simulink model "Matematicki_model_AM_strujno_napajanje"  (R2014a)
settings: Solver=ode3  StartTime=0.0  StopTime=Tfinalno  FixedStep=Tsim  RelTol=1e-3
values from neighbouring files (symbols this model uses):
  A1 = [-1/Tr 0; 0 -1/Tr]    [Matematicki_model_AM_strujno_napajanje_parametri.m]
  A2 = [0 1; -1 0]    [Matematicki_model_AM_strujno_napajanje_parametri.m]
  A3 = [0 -1; 1 0]    [Matematicki_model_AM_strujno_napajanje_parametri.m]
  Am = [-Kfv*p/J -Kel*p/J; 1 0]    [Matematicki_model_AM_strujno_napajanje_parametri.m]
  B = [Lm/Tr 0; 0 Lm/Tr]    [Matematicki_model_AM_strujno_napajanje_parametri.m]
  Bm = [p/J -p/J; 0 0]    [Matematicki_model_AM_strujno_napajanje_parametri.m]
  Im = sqrt(2)*Ieff    [Matematicki_model_AM_strujno_napajanje_parametri.m]
  Kp = -5.0    (= -5)    [Matematicki_model_AM_strujno_napajanje_parametri.m]
  Lm = 0.422    [Matematicki_model_AM_strujno_napajanje_parametri.m]
  Lr = Lxr+Lm    (= 0.462)    [Matematicki_model_AM_strujno_napajanje_parametri.m]
  Lsigma = Ls*sigm    (= 0.0765367965368)    [Matematicki_model_AM_strujno_napajanje_parametri.m]
  Mopt = 1    [Matematicki_model_AM_strujno_napajanje_parametri.m]
  p = 2    [Matematicki_model_AM_strujno_napajanje_parametri.m]
  Rs = 10.0    (= 10)    [Matematicki_model_AM_strujno_napajanje_parametri.m]
  Tn = 10*Tr    (= 0.733333333333)    [Matematicki_model_AM_strujno_napajanje_parametri.m]
  topt = 0    [Matematicki_model_AM_strujno_napajanje_parametri.m]
  TROUGAO_ZVEZDA = 0    [Matematicki_model_AM_strujno_napajanje_parametri.m]
  Tsim = Tpwm/16    (= 3.125e-06)    [Matematicki_model_AM_strujno_napajanje_parametri.m]
  wk = 1/Tr    (= 13.6363636364)    [Matematicki_model_AM_strujno_napajanje_parametri.m]
  wref = ws    [Matematicki_model_AM_strujno_napajanje_parametri.m]
  ws = 2*pi()*fs    [Matematicki_model_AM_strujno_napajanje_parametri.m]
libraries: simulink x1

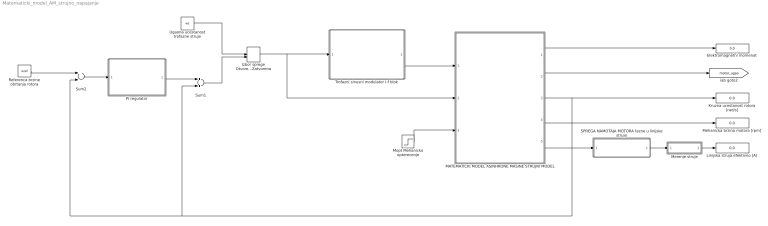
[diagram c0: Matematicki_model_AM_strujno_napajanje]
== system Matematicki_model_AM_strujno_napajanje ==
  Elektromagnetni momenat : Display
  Izbor sprege Otvorena / Zatvorena : ManualSwitch  CurrentSetting=0
  Kruzna ucestanost rotora [rad/s] : Display
  Linijska struja efektivno [A] : Display
  MATEMATICKI MODEL ASINHRONE MASINE STRUJNI MODEL : Subsystem
  Mehanicka brzina motora [rpm] : Display
  Merenje struje : Subsystem
  Mopt Mehanicko opterecenje : Step  Time=topt  After=Mopt  SampleTime=Tsim
  PI regulator : Subsystem
  Referenca brzine obrtanja rotora : Constant  Value=wref  SampleTime=Tsim
  SPREGA NAMOTAJA MOTORA fazne u linijske struje : Subsystem
  Sum1 : Sum  SampleTime=Tsim
  Sum2 : Sum  Inputs=+-  SampleTime=Tsim
  Trofazni sinusni modulator I-f blok : Subsystem
  Ugaona ucestanost trofazne struje : Constant  Value=ws  SampleTime=Tsim
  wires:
  Merenje struje/1(Is_eff) -> Linijska struja efektivno [A]/1
  SPREGA NAMOTAJA MOTORA fazne u linijske struje/1("Is_abc invertor ") -> Merenje struje/1(Is_abc)
  MATEMATICKI MODEL ASINHRONE MASINE STRUJNI MODEL/5(" Is_abc ") -> SPREGA NAMOTAJA MOTORA fazne u linijske struje/1(Is_abc fazno)
  MATEMATICKI MODEL ASINHRONE MASINE STRUJNI MODEL/4(Brzina meh [o/min]) -> Mehanicka brzina motora [rpm]/1
  MATEMATICKI MODEL ASINHRONE MASINE STRUJNI MODEL/1(M_el) -> Elektromagnetni momenat/1
  MATEMATICKI MODEL ASINHRONE MASINE STRUJNI MODEL/3(wr_el) -> Kruzna ucestanost rotora [rad/s]/1, Sum2/2, Sum1/2
  Referenca brzine obrtanja rotora/1 -> Sum2/1
  Sum2/1 -> PI regulator/1(e)
  PI regulator/1(wk) -> Sum1/1
  Trofazni sinusni modulator I-f blok/1(PWM) -> MATEMATICKI MODEL ASINHRONE MASINE STRUJNI MODEL/1(Is_abc)
  Izbor sprege Otvorena / Zatvorena/1 -> MATEMATICKI MODEL ASINHRONE MASINE STRUJNI MODEL/2(W_dq), Trofazni sinusni modulator I-f blok/1(ws)
  Sum1/1 -> Izbor sprege Otvorena / Zatvorena/2
  Ugaona ucestanost trofazne struje/1 -> Izbor sprege Otvorena / Zatvorena/1
  MATEMATICKI MODEL ASINHRONE MASINE STRUJNI MODEL/2(ugao rot_el) -> [motor_ugao]
  Mopt Mehanicko opterecenje/1 -> MATEMATICKI MODEL ASINHRONE MASINE STRUJNI MODEL/3(Mopt)

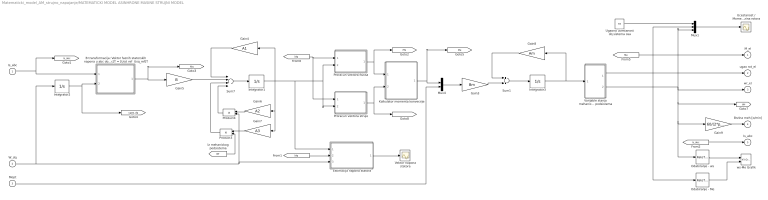
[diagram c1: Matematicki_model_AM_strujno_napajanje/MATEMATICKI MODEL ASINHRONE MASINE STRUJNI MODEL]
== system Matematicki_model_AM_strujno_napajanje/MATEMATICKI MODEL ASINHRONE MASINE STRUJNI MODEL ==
  Is_abc : Inport
  W_dq : Inport  Port=2
  Mopt : Inport  Port=3
  B transformacija: Vektor faznih statorskih napona u abc domenu u vektor napona u dq referentnom sistemu - [Usa  Usb Usc]T = [Usd_ref  Usq_ref]T : Subsystem
  Estimacija napona statora : Subsystem
  Gain3 : Gain  Gain=Bm  Multiplication=Matrix(K*u) (u vector)  SampleTime=Tsim
  Gain4 : Gain  Gain=A1  Multiplication=Matrix(K*u) (u vector)  SampleTime=Tsim
  Gain5 : Gain  Gain=B  Multiplication=Matrix(K*u) (u vector)  SampleTime=Tsim
  Gain6 : Gain  Gain=A2  Multiplication=Matrix(K*u) (u vector)  SampleTime=Tsim
  Gain7 : Gain  Gain=A3  Multiplication=Matrix(K*u) (u vector)  SampleTime=Tsim
  Gain8 : Gain  Gain=Am  Multiplication=Matrix(K*u) (u vector)  SampleTime=Tsim
  Gain9 : Gain  Gain=60/(2*pi()*p)  SampleTime=Tsim
  Integrator1 : Integrator  InitialCondition=[0,0]
  Integrator2 : Integrator
  Integrator3 : Integrator  InitialCondition=[0,0]
  Kalkulator momenta konverzije : Subsystem
  Mux1 : Mux  Inputs=3
  Mux4 : Mux  Inputs=2
  Odabiranje - Me : RateTransition  OutPortSampleTime=100*Tsim
  Odabiranje - ws : RateTransition  OutPortSampleTime=100*Tsim
  Product3 : Product  SampleTime=Tsim
  Product4 : Product  SampleTime=Tsim
  Proracun vektora fluksa : Subsystem
  Proracun vektora struje : Subsystem
  Sum1 : Sum  SampleTime=Tsim
  Sum7 : Sum  Inputs=++++  SampleTime=Tsim
  Ucestanost / Momenat / Brzina rotora : Scope
  Ugaona ucestanost dq sistema osa : Constant  Value=ws  SampleTime=Tsim
  Varijable stanja mehanickog podsistema : Subsystem
  Vektor napona statora : Scope
  ws-Me Grafik : simulink/Sinks/XY Graph  xmin=-400  xmax=400  ymin=-5  ymax=5  st=100*Tsim
  M_el : Outport  InitialOutput=0
  ugao rot_el : Outport  Port=2  InitialOutput=0
  wr_el : Outport  Port=3  InitialOutput=0
  Brzina meh [o/min] : Outport  Port=4  InitialOutput=0
  " Is_abc " : Outport  Port=5  InitialOutput=0
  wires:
  Odabiranje - Me/1 -> ws-Me Grafik/2
  Odabiranje - ws/1 -> ws-Me Grafik/1
  Mux1/1 -> Ucestanost / Momenat / Brzina rotora/1
  [Is_abc] -> " Is_abc "/1
  Integrator3/1 -> Gain8/1, Varijable stanja mehanickog podsistema/1(X2)
  Gain8/1 -> Sum1/1
  Sum1/1 -> Integrator3/1
  Gain3/1 -> Sum1/2
  Mux4/1 -> Gain3/1
  Gain9/1 -> Brzina meh [o/min]/1
  Varijable stanja mehanickog podsistema/2(w) -> Odabiranje - ws/1, Gain9/1, [Wr], Mux1/3, wr_el/1
  Varijable stanja mehanickog podsistema/1(theta) -> ugao rot_el/1
  [Me] -> Odabiranje - Me/1, Mux1/2, M_el/1
  Mopt/1 -> Mux4/2
  Kalkulator momenta konverzije/1(Me) -> Mux4/1, [Me]
  Proracun vektora struje/1(I) -> Kalkulator momenta konverzije/2(I), [I]
  Proracun vektora fluksa/1(PSI) -> Kalkulator momenta konverzije/1(PSI), [PSI]
  Product4/1 -> Sum7/4
  W_dq/1 -> Product4/2, Estimacija napona statora/3(wdq), Integrator2/1
  Gain5/1 -> Sum7/2
  Gain4/1 -> Sum7/1
  Sum7/1 -> Integrator1/1
  Gain6/1 -> Product4/1
  Gain7/1 -> Product3/1
  Product3/1 -> Sum7/3
  [Wr] -> Product3/2
  Is_abc/1 -> [Is_abc], B transformacija: Vektor faznih statorskih napona u abc domenu u vektor napona u dq referentnom sistemu - [Usa  Usb Usc]T = [Usd_ref  Usq_ref]T/1(Is_abc)
  [Idq] -> Proracun vektora fluksa/1(Is), Proracun vektora struje/1(Is)
  Estimacija napona statora/1(Vs) -> Vektor napona statora/1
  Integrator2/1 -> [ugao_dq], B transformacija: Vektor faznih statorskih napona u abc domenu u vektor napona u dq referentnom sistemu - [Usa  Usb Usc]T = [Usd_ref  Usq_ref]T/2(ugao_dq)
  B transformacija: Vektor faznih statorskih napona u abc domenu u vektor napona u dq referentnom sistemu - [Usa  Usb Usc]T = [Usd_ref  Usq_ref]T/1(Is_dq) -> Gain5/1, [Idq]
  [Idq] -> Estimacija napona statora/2(Is)
  Integrator1/1 -> Gain6/1, Gain7/1, Estimacija napona statora/1(PSIr), Proracun vektora struje/2(PSIr), Proracun vektora fluksa/2(PSIr), Gain4/1
  Ugaona ucestanost dq sistema osa/1 -> Mux1/1

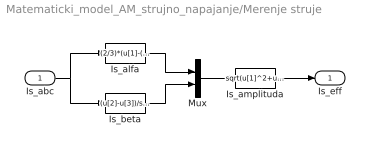
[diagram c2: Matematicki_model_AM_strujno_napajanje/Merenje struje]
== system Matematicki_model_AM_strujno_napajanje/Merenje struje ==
  Is_abc : Inport
  Is_alfa : Fcn  Expr=(2/3)*(u[1]-(u[2]+u[3])/2)  SampleTime=Tsim
  Is_amplituda : Fcn  Expr=sqrt(u[1]^2+u[2]^2)/sqrt(2)  SampleTime=Tsim
  Is_beta : Fcn  Expr=(u[2]-u[3])/sqrt(3)  SampleTime=Tsim
  Mux : Mux  Inputs=2
  Is_eff : Outport
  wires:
  Is_abc/1 -> Is_beta/1, Is_alfa/1
  Is_alfa/1 -> Mux/1
  Is_beta/1 -> Mux/2
  Mux/1 -> Is_amplituda/1
  Is_amplituda/1 -> Is_eff/1

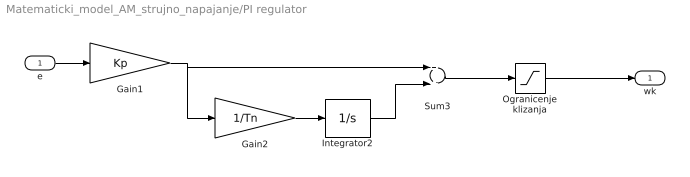
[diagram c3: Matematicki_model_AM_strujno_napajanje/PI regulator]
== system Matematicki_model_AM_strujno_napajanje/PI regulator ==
  e : Inport
  Gain1 : Gain  Gain=Kp  SampleTime=Tsim
  Gain2 : Gain  Gain=1/Tn  SampleTime=Tsim
  Integrator2 : Integrator  InitialCondition=[0]
  Ogranicenje klizanja : Saturate  UpperLimit=inf  LowerLimit=wk  SampleTime=Tsim
  Sum3 : Sum  SampleTime=Tsim
  wk : Outport
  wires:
  Gain1/1 -> Sum3/1, Gain2/1
  e/1 -> Gain1/1
  Sum3/1 -> Ogranicenje klizanja/1
  Integrator2/1 -> Sum3/2
  Gain2/1 -> Integrator2/1
  Ogranicenje klizanja/1 -> wk/1

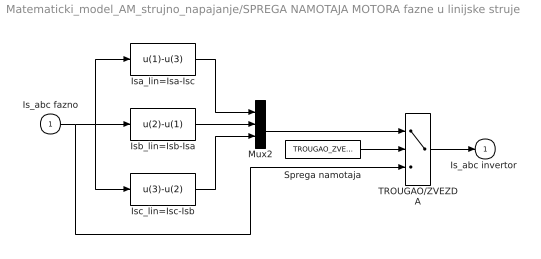
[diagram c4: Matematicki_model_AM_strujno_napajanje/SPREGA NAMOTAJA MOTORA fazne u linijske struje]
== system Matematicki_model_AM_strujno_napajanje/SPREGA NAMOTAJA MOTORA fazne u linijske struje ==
  Is_abc fazno : Inport
  Isa_lin=Isa-Isc : Fcn  Expr=u(1)-u(3)  SampleTime=Tsim
  Isb_lin=Isb-Isa : Fcn  Expr=u(2)-u(1)  SampleTime=Tsim
  Isc_lin=Isc-Isb : Fcn  Expr=u(3)-u(2)  SampleTime=Tsim
  Mux2 : Mux  Inputs=3
  Sprega namotaja : Constant  Value=TROUGAO_ZVEZDA
  TROUGAO/ZVEZDA : Switch  Threshold=0.1  SampleTime=Tsim
  "Is_abc invertor " : Outport  InitialOutput=0
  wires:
  Sprega namotaja/1 -> TROUGAO/ZVEZDA/2
  Mux2/1 -> TROUGAO/ZVEZDA/1
  TROUGAO/ZVEZDA/1 -> "Is_abc invertor "/1
  Is_abc fazno/1 -> TROUGAO/ZVEZDA/3, Isa_lin=Isa-Isc/1, Isb_lin=Isb-Isa/1, Isc_lin=Isc-Isb/1
  Isa_lin=Isa-Isc/1 -> Mux2/1
  Isb_lin=Isb-Isa/1 -> Mux2/2
  Isc_lin=Isc-Isb/1 -> Mux2/3

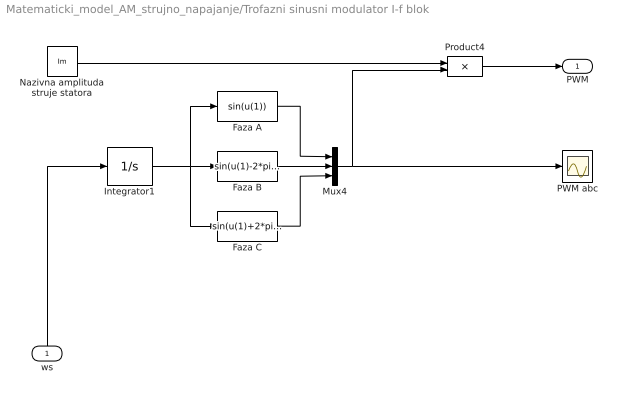
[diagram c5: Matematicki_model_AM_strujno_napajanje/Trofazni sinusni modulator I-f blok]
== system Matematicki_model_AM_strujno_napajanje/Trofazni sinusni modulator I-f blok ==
  ws : Inport
  Faza A : Fcn  Expr=sin(u(1))  SampleTime=Tsim
  Faza B : Fcn  Expr=sin(u(1)-2*pi()/3)  SampleTime=Tsim
  Faza C : Fcn  Expr=sin(u(1)+2*pi()/3)  SampleTime=Tsim
  Integrator1 : Integrator  InitialCondition=[0]
  Mux4 : Mux  Inputs=3
  Nazivna amplituda struje statora : Constant  Value=Im  SampleTime=Tsim
  PWM abc : Scope
  Product4 : Product  SampleTime=Tsim
  PWM : Outport
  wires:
  Faza B/1 -> Mux4/2
  Faza A/1 -> Mux4/1
  Faza C/1 -> Mux4/3
  Mux4/1 -> Product4/2, PWM abc/1
  Nazivna amplituda struje statora/1 -> Product4/1
  Product4/1 -> PWM/1
  ws/1 -> Integrator1/1
  Integrator1/1 -> Faza C/1, Faza B/1, Faza A/1

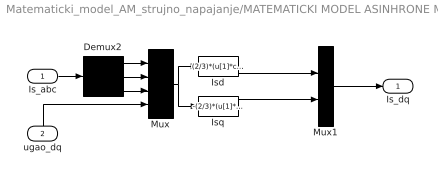
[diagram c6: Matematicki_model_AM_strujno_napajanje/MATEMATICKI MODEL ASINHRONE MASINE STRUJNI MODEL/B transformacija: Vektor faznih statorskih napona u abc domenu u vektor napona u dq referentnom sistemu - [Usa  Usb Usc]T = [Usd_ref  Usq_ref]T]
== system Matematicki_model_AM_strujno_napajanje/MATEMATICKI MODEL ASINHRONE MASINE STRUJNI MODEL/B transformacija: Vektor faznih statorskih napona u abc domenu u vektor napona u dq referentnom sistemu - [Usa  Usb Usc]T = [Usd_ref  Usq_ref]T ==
  Is_abc : Inport
  ugao_dq : Inport  Port=2
  Demux2 : Demux  Outputs=3
  Isd : Fcn  Expr=(2/3)*(u[1]*cos(u[4])+u[2]*cos(u[4]-2*pi/3)+u[3]*cos(u[4]-4*pi/3))  SampleTime=Tsim
  Isq : Fcn  Expr=-(2/3)*(u[1]*sin(u[4])+u[2]*sin(u[4]-2*pi/3)+u[3]*sin(u[4]-4*pi/3))  SampleTime=Tsim
  Mux : Mux
  Mux1 : Mux  Inputs=2
  Is_dq : Outport
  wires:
  Mux1/1 -> Is_dq/1
  Is_abc/1 -> Demux2/1
  ugao_dq/1 -> Mux/4
  Demux2/1 -> Mux/1
  Demux2/3 -> Mux/3
  Demux2/2 -> Mux/2
  Mux/1 -> Isd/1, Isq/1
  Isq/1 -> Mux1/2
  Isd/1 -> Mux1/1

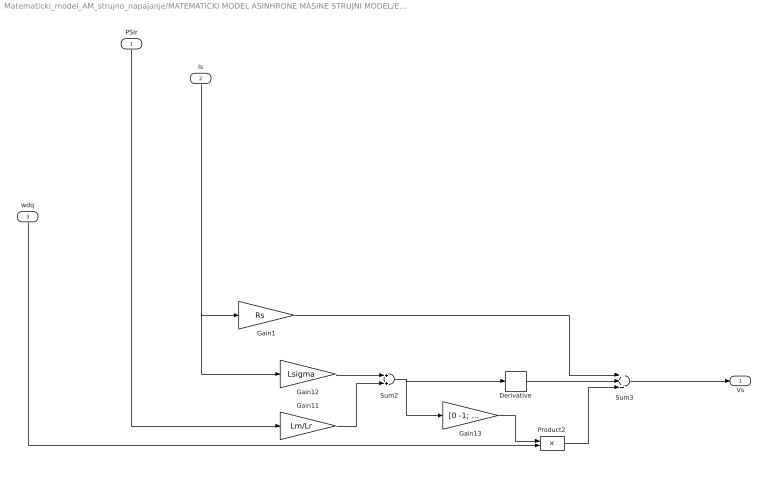
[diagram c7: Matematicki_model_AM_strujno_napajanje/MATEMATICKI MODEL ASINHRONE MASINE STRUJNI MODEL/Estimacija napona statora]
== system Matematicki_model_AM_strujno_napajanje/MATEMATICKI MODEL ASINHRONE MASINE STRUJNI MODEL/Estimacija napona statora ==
  PSIr : Inport
  Is : Inport  Port=2
  wdq : Inport  Port=3
  Derivative : Derivative
  Gain1 : Gain  Gain=Rs  SampleTime=Tsim
  Gain11 : Gain  Gain=Lm/Lr  SampleTime=Tsim
  Gain12 : Gain  Gain=Lsigma  SampleTime=Tsim
  Gain13 : Gain  Gain=[0 -1; 1 0]  Multiplication=Matrix(K*u) (u vector)  SampleTime=Tsim
  Product2 : Product  SampleTime=Tsim
  Sum2 : Sum  SampleTime=Tsim
  Sum3 : Sum  Inputs=+++  SampleTime=Tsim
  Vs : Outport
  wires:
  Gain11/1 -> Sum2/2
  Gain12/1 -> Sum2/1
  Sum2/1 -> Gain13/1, Derivative/1
  Product2/1 -> Sum3/3
  Sum3/1 -> Vs/1
  Gain1/1 -> Sum3/1
  Derivative/1 -> Sum3/2
  Gain13/1 -> Product2/1
  wdq/1 -> Product2/2
  PSIr/1 -> Gain11/1
  Is/1 -> Gain12/1, Gain1/1

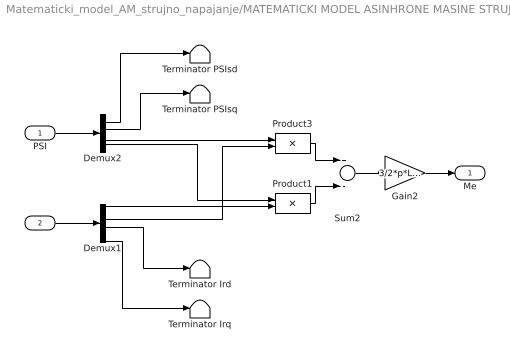
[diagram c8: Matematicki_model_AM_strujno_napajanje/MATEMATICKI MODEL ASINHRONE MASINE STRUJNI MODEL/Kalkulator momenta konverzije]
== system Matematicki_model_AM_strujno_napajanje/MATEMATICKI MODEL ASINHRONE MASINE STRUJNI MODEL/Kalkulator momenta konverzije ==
  PSI : Inport
  I : Inport  Port=2
  Demux1 : Demux
  Demux2 : Demux
  Gain2 : Gain  Gain=3/2*p*Lm/Lr  SampleTime=Tsim
  Product1 : Product  SampleTime=Tsim
  Product3 : Product  SampleTime=Tsim
  Sum2 : Sum  Inputs=+-  SampleTime=Tsim
  Terminator Ird : Terminator
  Terminator Irq : Terminator
  Terminator PSIsd : Terminator
  Terminator PSIsq : Terminator
  Me : Outport
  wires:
  Demux1/4 -> Terminator Irq/1
  Demux1/3 -> Terminator Ird/1
  Sum2/1 -> Gain2/1
  Gain2/1 -> Me/1
  Product1/1 -> Sum2/2
  Product3/1 -> Sum2/1
  Demux2/3 -> Product3/1
  Demux2/4 -> Product1/1
  I/1 -> Demux1/1
  Demux1/2 -> Product3/2
  Demux1/1 -> Product1/2
  Demux2/2 -> Terminator PSIsq/1
  Demux2/1 -> Terminator PSIsd/1
  PSI/1 -> Demux2/1

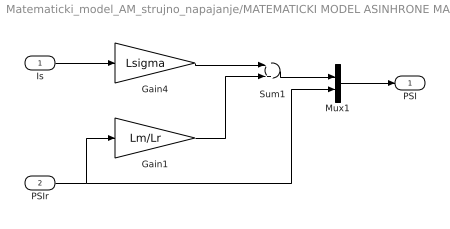
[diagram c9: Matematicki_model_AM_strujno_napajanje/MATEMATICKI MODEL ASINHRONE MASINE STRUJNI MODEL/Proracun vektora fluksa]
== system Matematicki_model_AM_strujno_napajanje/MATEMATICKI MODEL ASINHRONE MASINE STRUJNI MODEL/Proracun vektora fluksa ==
  Is : Inport
  PSIr : Inport  Port=2
  Gain1 : Gain  Gain=Lm/Lr  SampleTime=Tsim
  Gain4 : Gain  Gain=Lsigma  SampleTime=Tsim
  Mux1 : Mux  Inputs=2
  Sum1 : Sum  SampleTime=Tsim
  PSI : Outport
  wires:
  Sum1/1 -> Mux1/1
  Gain4/1 -> Sum1/1
  Gain1/1 -> Sum1/2
  PSIr/1 -> Mux1/2, Gain1/1
  Mux1/1 -> PSI/1
  Is/1 -> Gain4/1

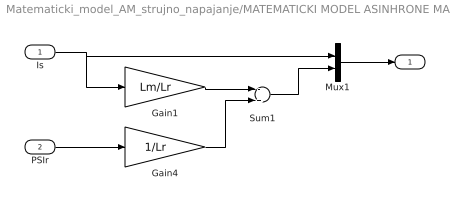
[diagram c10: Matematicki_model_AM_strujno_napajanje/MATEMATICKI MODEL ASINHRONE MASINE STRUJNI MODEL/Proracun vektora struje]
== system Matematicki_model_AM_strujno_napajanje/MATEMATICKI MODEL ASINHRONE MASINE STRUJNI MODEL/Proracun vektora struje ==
  Is : Inport
  PSIr : Inport  Port=2
  Gain1 : Gain  Gain=Lm/Lr  SampleTime=Tsim
  Gain4 : Gain  Gain=1/Lr  SampleTime=Tsim
  Mux1 : Mux  Inputs=2
  Sum1 : Sum  Inputs=-+  SampleTime=Tsim
  I : Outport
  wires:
  Sum1/1 -> Mux1/2
  Gain4/1 -> Sum1/2
  Gain1/1 -> Sum1/1
  PSIr/1 -> Gain4/1
  Mux1/1 -> I/1
  Is/1 -> Mux1/1, Gain1/1

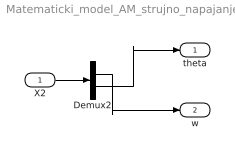
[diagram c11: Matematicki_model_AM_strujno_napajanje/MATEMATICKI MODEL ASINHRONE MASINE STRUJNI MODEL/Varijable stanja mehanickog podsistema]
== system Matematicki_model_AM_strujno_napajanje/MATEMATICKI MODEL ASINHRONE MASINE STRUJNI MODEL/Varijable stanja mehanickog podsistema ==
  X2 : Inport
  Demux2 : Demux  Outputs=2
  theta : Outport
  w : Outport  Port=2
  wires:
  Demux2/1 -> w/1
  Demux2/2 -> theta/1
  X2/1 -> Demux2/1
